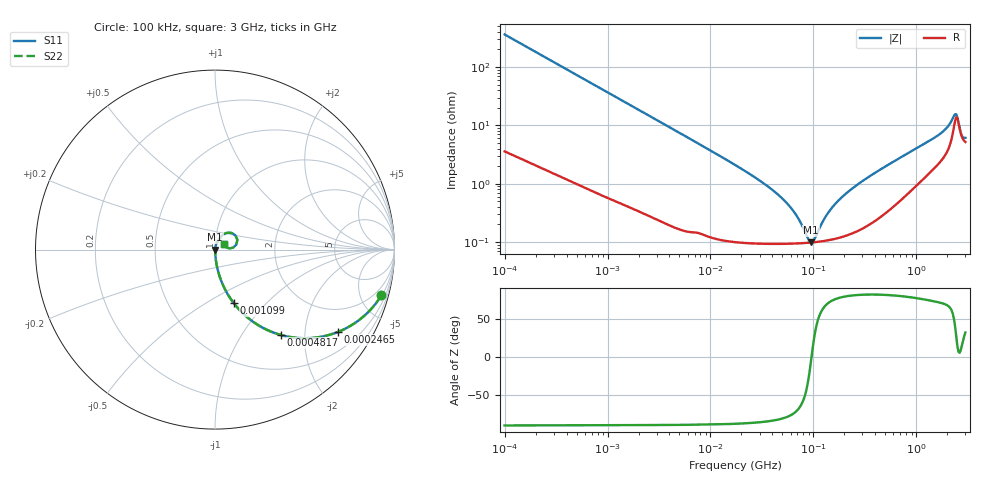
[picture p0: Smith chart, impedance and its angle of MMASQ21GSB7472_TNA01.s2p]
! MMASQ21GSB7472_TNA01  S-PARAMETER MODEL  ( Standard Model )
! Model Generated by TAIYO YUDEN Corporation (http://www.ty-top.com)
! Version 1.0
! TAIYO YUDEN Control No. 220601
! Copyright(c) 2013 TAIYO YUDEN CO.,LTD. All Rights Reserved.
! Product Description (link to TY-COMPAS)
! https://ds.yuden.co.jp/TYCOMPAS/or/detail?pn=MMASQ21GSB7472KTNA01&u=M
! Products Name : Multilayer Ceramic Capacitors
! Characteristics :
!  Capacitance : 4700 [pF] , Rated Voltage : 250 [V] , TCC : X7R
!  Case Size : 2.0 x 1.25 / 0.079 x 0.049 [mm/inch] , Thickness : 1.25 / 0.049 [mm/inch]
!  (Conditions: Temperature = 25 [degC] , DC Bias Voltage = 0 [V])
! External Node Assignments :
!  1  o---| |---o  2
! GND o---------o GND
! Frequency Range : 100kHz  -  3GHz  [ 401 STEP ]
# MHZ S RI R 50
! Freq[MHz].  S11 Real  S11 Imag  S21 Real  S21 Imag  S12 Real  S12 Imag  S22 Real  S22 Imag
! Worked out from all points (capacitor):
!   401 points, 100 kHz to 3 GHz, reference 50 ohm
!   read as one part in series: C = 4.39 nF near 105.3 kHz
!   lowest |Z| = 98.4 mohm at 94.9 MHz (marker M1)
!   series resonance near 95.95 MHz, so ESL is about 630 pH
!   S11 on the Smith chart (normalised r, x): 100 kHz: 1.07, -7.23; 246.5 kHz: 1.03, -2.95; 481.7 kHz: 1.02, -1.52; 1.099 MHz: 1.01, -0.67; 3 GHz: 1.10, +0.06
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0.1  0.9268 -0.2555  0.0732 0.2555  0.0732 0.2555  0.9268 -0.2555
0.159027  0.8361 -0.3648  0.1639 0.3648  0.1639 0.3648  0.8361 -0.3648
0.246461  0.6835 -0.4593  0.3165 0.4593  0.3165 0.4593  0.6835 -0.4593
0.481683  0.3674 -0.4755  0.6326 0.4755  0.6326 0.4755  0.3674 -0.4755
0.562235  0.3004 -0.4516  0.6996 0.4516  0.6996 0.4516  0.3004 -0.4516
1.09883  0.1048 -0.2984  0.8952 0.2984  0.8952 0.2984  0.1048 -0.2984
3.161081  0.0159 -0.1155  0.9841 0.1155  0.9841 0.1155  0.0159 -0.1155
17.7727  0.00141 -0.0204  0.9986 0.0204  0.9986 0.0204  0.00141 -0.0204
34.73492  0.00102 -0.0094  0.999 0.0094  0.999 0.0094  0.00102 -0.0094
52.46276  0.000955 -0.00502  0.999 0.00502  0.999 0.00502  0.000955 -0.00502
67.88584  0.00095 -0.00276  0.999 0.00276  0.999 0.00276  0.00095 -0.00276
94.90424  0.000979 -8.55e-05  0.999 8.55e-05  0.999 8.55e-05  0.000979 -8.55e-05
97.38194  0.000983 0.000116  0.999 -0.000116  0.999 -0.000116  0.000983 0.000116
132.6759  0.00106 0.00258  0.9989 -0.00258  0.9989 -0.00258  0.00106 0.00258
176.1623  0.0012 0.00505  0.9988 -0.00505  0.9988 -0.00505  0.0012 0.00505
273.0175  0.00165 0.00972  0.9983 -0.00972  0.9983 -0.00972  0.00165 0.00972
547.5153  0.00396 0.0213  0.996 -0.0213  0.996 -0.0213  0.00396 0.0213
1658.39  0.0258 0.0624  0.9742 -0.0624  0.9742 -0.0624  0.0258 0.0624
2378.954  0.1128 0.0801  0.8872 -0.0801  0.8872 -0.0801  0.1128 0.0801
2504.792  0.1186 0.0269  0.8814 -0.0269  0.8814 -0.0269  0.1186 0.0269
2776.789  0.0601 0.0153  0.9399 -0.0153  0.9399 -0.0153  0.0601 0.0153
3000  0.0502 0.0292  0.9498 -0.0292  0.9498 -0.0292  0.0502 0.0292
